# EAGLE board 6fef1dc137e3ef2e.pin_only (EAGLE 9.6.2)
REV: B

Size 33.02 x 17.78 mm. Coordinates in mm from the lower left corner, seen from the top.
Outline: 0,17.78 0,0 33.02,0 33.02,17.78 0,17.78
Copper layers (1*16): Top 0.035mm / dielectric 1.5mm / Bottom 0.035mm
Design rules "adafruit 7-7 *": minimum track width 7mil, minimum drill 15.5mil, track to track 8mil, track to pad 7mil, pad to pad 7mil, via to via 7mil, smd to smd 7mil, copper to edge 10mil, drill to drill 8mil, minimum pad ring 10mil, minimum via ring 8mil, stop-mask expansion 2mil, vias tented up to drill 20mil, thermal gap 10mil
Net classes: 1 power: width 0.203 mm

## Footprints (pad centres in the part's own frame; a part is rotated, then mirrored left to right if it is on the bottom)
_0805MP = smd 1.2 x 1.3: 1 -1.016,0; 2 1.016,0
_0402NO = smd 0.6 x 0.6: 1 -0.508,0; 2 0.508,0
_0603MP = smd 0.8 x 0.8: 1 -0.762,0; 2 0.762,0
0603-NO = smd 1.075 x 1: 1 -0.85,0; 2 0.85,0
JST_SH4_SKINNY = smd 0.5 x 1.55: 1 -1.5,2.514; 2 -0.5,2.514; 3 0.5,2.514; 4 1.5,2.514 | smd 1.2 x 1.8: MT1 -2.8,-1.386; MT2 2.8,-1.386
SOD-323F = smd 1 x 0.8: A -1,0; C 1,0
CHIPLED_0603_NOOUTLINE = smd 0.8 x 0.8: A 0,-0.75; C 0,0.75
QFN56_7MM_REDUCEDEPAD = smd 0.875 x 0.2: 1 -3.45,2.6; 2 -3.45,2.2; 3 -3.45,1.8; 4 -3.45,1.4; 5 -3.45,1; 6 -3.45,0.6; 7 -3.45,0.2; 8 -3.45,-0.2; 9 -3.45,-0.6; 10 -3.45,-1; 11 -3.45,-1.4; 12 -3.45,-1.8; 13 -3.45,-2.2; 14 -3.45,-2.6; 29 3.45,-2.6; 30 3.45,-2.2; 31 3.45,-1.8; 32 3.45,-1.4; 33 3.45,-1; 34 3.45,-0.6; 35 3.45,-0.2; 36 3.45,0.2; 37 3.45,0.6; 38 3.45,1; 39 3.45,1.4; 40 3.45,1.8; 41 3.45,2.2; 42 3.45,2.6 | smd 0.2 x 0.875: 15 -2.6,-3.45; 16 -2.2,-3.45; 17 -1.8,-3.45; 18 -1.4,-3.45; 19 -1,-3.45; 20 -0.6,-3.45; 21 -0.2,-3.45; 22 0.2,-3.45; 23 0.6,-3.45; 24 1,-3.45; 25 1.4,-3.45; 26 1.8,-3.45; 27 2.2,-3.45; 28 2.6,-3.45; 43 2.6,3.45; 44 2.2,3.45; 45 1.8,3.45; 46 1.4,3.45; 47 1,3.45; 48 0.6,3.45; 49 0.2,3.45; 50 -0.2,3.45; 51 -0.6,3.45; 52 -1,3.45; 53 -1.4,3.45; 54 -1.8,3.45; 55 -2.2,3.45; 56 -2.6,3.45 | smd 3.2 x 3.2: P$1 0,0
1X13_CASTEL = drill 1 pad 1.778: 1 -15.24,0; 2 -12.7,0; 3 -10.16,0; 4 -7.62,0; 5 -5.08,0; 6 -2.54,0; 7 0,0; 8 2.54,0; 9 5.08,0; 10 7.62,0; 11 10.16,0; 12 12.7,0; 13 15.24,0 | drill 1.397 pad 1.778 long: 1C -15.24,-1.524; 2C -12.7,-1.524; 3C -10.16,-1.524; 4C -7.62,-1.524; 5C -5.08,-1.524; 6C -2.54,-1.524; 7C 0,-1.524; 8C 2.54,-1.524; 9C 5.08,-1.524; 10C 7.62,-1.524; 11C 10.16,-1.524; 12C 12.7,-1.524; 13C 15.24,-1.524
SK6805_1515 = smd 0.5 x 0.5: 1 -0.5,-0.45; 2 0.5,-0.45; 3 0.5,0.45; 4 -0.5,0.45
0805-NO = smd 1.24 x 1.5: 1 -0.95,0; 2 0.95,0
SOLDERJUMPER_ARROW_NOPASTE = smd 0.762 x 1.524: 1 -1.016,0; 2 1.016,0
BTN_KMR2_4.6X2.8 = smd 0.9 x 0.9: A 2.05,0.8; A' -2.05,0.8; B 2.05,-0.8; B' -2.05,-0.8
TESTPOINT_ROUND_1.5MM_NO = smd 1.5 x 1.5: P$1 0,0
SOT23-5 = smd 0.55 x 1.2: 1 -0.95,-1.3; 2 0,-1.3; 3 0.95,-1.3; 4 0.95,1.3; 5 -0.95,1.3
USON8_4X4 = smd 0.6 x 0.4: 1 -1.85,1.2; 2 -1.85,0.4; 3 -1.85,-0.4; 4 -1.85,-1.2; 5 1.85,-1.2; 6 1.85,-0.4; 7 1.85,0.4; 8 1.85,1.2 | smd 2 x 3: PAD 0,0
FIDUCIAL_1MM = smd 1 x 1: 1 0,0
USB_C_CUSB31-CFM2AX-01-X = smd 0.575 x 1.15: A1B12 -3.2,3.545; A4B9 -2.4,3.545; B1A12 3.2,3.545; B4A9 2.4,3.545 | smd 0.275 x 1.15: A5 -1.25,3.545; A6 -0.25,3.545; A7 0.25,3.545; A8 1.25,3.545; B5 1.75,3.545; B6 0.75,3.545; B7 -0.75,3.545; B8 -1.75,3.545 | drill 0.6 pad 1 long: M1 -4.32,2.97; M2 4.32,2.97; M3 -4.32,-1.21; M4 4.32,-1.21 | hole 0.65: 2.89,2.47; -2.89,2.47
CRYSTAL_2.5X2 = smd 0.9 x 0.75: 1 -0.825,-0.625; 2 0.825,-0.625; 3 0.825,0.625; 4 -0.825,0.625

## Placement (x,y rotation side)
C6  10µF  [_0805MP]  8.66,13.8 0 top
C7  0.1uF  [_0402NO]  14.29,12.76 270 top
C8  10µF  [_0805MP]  11.24,9.84 90 top
C9  0.1uF  [_0402NO]  25.53,10.29 0 top
C10  1uF  [_0603MP]  12.18,13.7 180 top
C11  0.1uF  [_0402NO]  25.23,11.18 180 top
C12  1uF  [_0603MP]  12.18,12.17 180 top
C13  0.1uF  [_0402NO]  15.44,3.56 270 top
C14  0.1uF  [_0402NO]  19.44,13.72 180 top
C15  1uF  [0603-NO]  9.59,6.03 270 top
C16  0.1uF  [_0402NO]  21.08,3.67 0 top
C17  0.1uF  [_0402NO]  16.05,14.14 180 top
C19  22pF  [_0402NO]  24.51,5.97 180 top
C20  22pF  [_0402NO]  26.61,5.97 0 top
CONN1  STEMMA_I2C_QTSKINNY  [JST_SH4_SKINNY]  30.48,8.89 90 top
D1  NSR0320  [SOD-323F]  8.76,8.32 0 top
D2  GREEN  [CHIPLED_0603_NOOUTLINE]  1.46,14.35 270 top
D3  NSR0320  [SOD-323F]  25.93,3.85 0 top
IC2  RP2040_QFN56  [QFN56_7MM_REDUCEDEPAD]  19.37,9.18 90 top
JP1  [1X13_CASTEL]  16.51,16.51 180 top
JP2  [1X13_CASTEL]  16.51,1.27 0 top
LED1  WS2812B_SK6805_1515  [SK6805_1515]  23.98,13.35 0 top
R1  5.1K  [_0402NO]  4.7,3.49 0 top
R2  5.1K  [_0402NO]  2.6,3.49 180 top
R3  27  [_0402NO]  13.97,10.19 180 top
R4  27  [_0402NO]  13.97,11.14 180 top
R5  10K  [_0402NO]  15.54,5.03 0 top
R6  1K  [_0402NO]  25.59,9.4 180 top
R7  10K  [_0402NO]  3.62,14.1 0 top
R8  FUSE  [0805-NO]  8,5.97 90 top
R9  10K  [_0402NO]  25.78,14.1 0 top
R10  5.1K  [_0402NO]  25.78,13.14 0 top
R11  1K  [_0402NO]  9.18,3.84 180 top
R12  5.1K  [_0402NO]  26.35,12.13 0 top
SJ1  [SOLDERJUMPER_ARROW_NOPASTE]  1.91,8.89 180 bottom
SW2  KMR2  [BTN_KMR2_4.6X2.8]  30.23,13.84 0 top
SW3  KMR2  [BTN_KMR2_4.6X2.8]  30.23,3.87 180 top
TP1  [TESTPOINT_ROUND_1.5MM_NO]  30.3,3.4 0 bottom
U2  AP2112K-3.3  [SOT23-5]  8.7,10.93 180 top
U5  8MB QSPI Flash  [USON8_4X4]  12.32,5.65 90 top
U$17  [KB2040_BOT]  0,17.78 180 bottom
U$19  [KB2040_TOP]  0,0 0 top
U$20  [PCBFEAT-REV-040]  25.27,8.7 180 bottom
U$34  FIDUCIAL_1MM  [FIDUCIAL_1MM]  30.8,13.64 270 top
U$35  FIDUCIAL_1MM  [FIDUCIAL_1MM]  0.99,11.03 270 top
X6  USB TYPE C  [USB_C_CUSB31-CFM2AX-01-X]  2.6,8.89 270 top
Y1  12MHZ  [CRYSTAL_2.5X2]  25.15,7.68 180 top

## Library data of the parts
C6 C7 C9-C17 C19 C20 CONN1 D2 JP1 JP2 LED1 R1-R12 SW2 SW3 TP1 U2 U5 Y1 = microbuilder
C8 = microbuilder; COMPANY: ADAFRUIT INDUSTRIES; DRAWN: KTOWN; REV: B
D1 D3 = adafruit
IC2 = adafruit_micro
SJ1 U$34 U$35 = microbuilder; BOM: EXCLUDE
U$17 U$19 = keeb_silks
U$20 = microbuilder; REV: B
X6 = adafruit_electromech

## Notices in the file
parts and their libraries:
microbuilder: This work is placed in the public domain, and may be freely used for commercial and non-commercial work with the following conditions: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
